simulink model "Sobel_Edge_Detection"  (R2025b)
settings: Solver=VariableStepAuto  StartTime=0.0  StopTime=inf  RelTol=1e-3  EnableMultiTasking=on
undefined symbols (not defined in the file or in its folder): True
libraries: visionsinks x2, dspvision x1

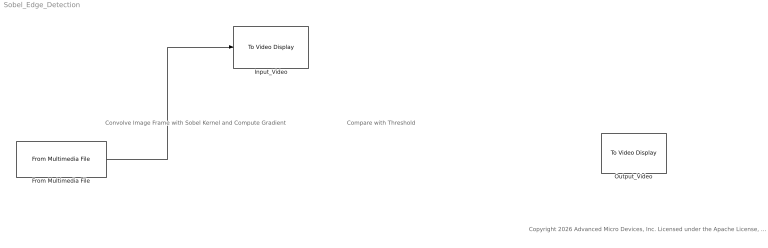
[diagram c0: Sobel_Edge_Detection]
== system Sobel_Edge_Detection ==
  note: Compare with Threshold
  note: Convolve Image Frame with Sobel Kernel and Compute Gradient
  note: Copyright 2026 Advanced Micro Devices, Inc. Licensed under the Apache License, Version 2.0 (the "License"); you may not use this file except in compliance with the License. You may obtain a copy of the License at http://www.apache.org/licenses/LICENSE-2.0 Unless required by applicable law or agreed to in writing, software distributed under the License is distributed on an "AS IS" BASIS, WITHOUT WARRANTIES OR CONDITIONS OF ANY KIND, either express or implied. See the License for the specific language governing permissions and limitations under the License.
  From Multimedia File : dspvision/From Multimedia File  inputFilename=visiontraffic.avi  readRange=[1 Inf]  loop=on  numPlays=inf  outputStreams=Video only  videoDataType=uint8  audioDataType=int16  inheritSampleTime=off  userDefinedSampleTime=1/30  noAudioOutput=off  isIntensityVideo=off  fourcc=Intensity  colorVideoFormat=One multidimensional signal  outputEOF=off  dataOrg=Column-major  audioFrameSize=1024  computeAudioFrameSize=off  outSamplingMode=Sample based
  Input_Video : visionsinks/To Video Display  windowSizeMode=True size (1:1)  openAtMdlStart=on  fullScreen=off  videoWindowX=197  videoWindowY=628  saveWindowSize=off  videoWindowWidth=160  videoWindowHeight=120  inputColorFormat=RGB  inputType=Obsolete  imagePorts=One multidimensional signal  OutputDevice=On-screen video monitor  dataOrg=Column-major  isWindowOpen=off
  Output_Video : visionsinks/To Video Display  windowSizeMode=True size (1:1)  openAtMdlStart=on  fullScreen=off  videoWindowX=1115  videoWindowY=603  saveWindowSize=off  videoWindowWidth=640  videoWindowHeight=360  inputColorFormat=RGB  inputType=Obsolete  imagePorts=One multidimensional signal  OutputDevice=On-screen video monitor  dataOrg=Column-major  isWindowOpen=off
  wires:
  From Multimedia File/1 -> Input_Video/1
